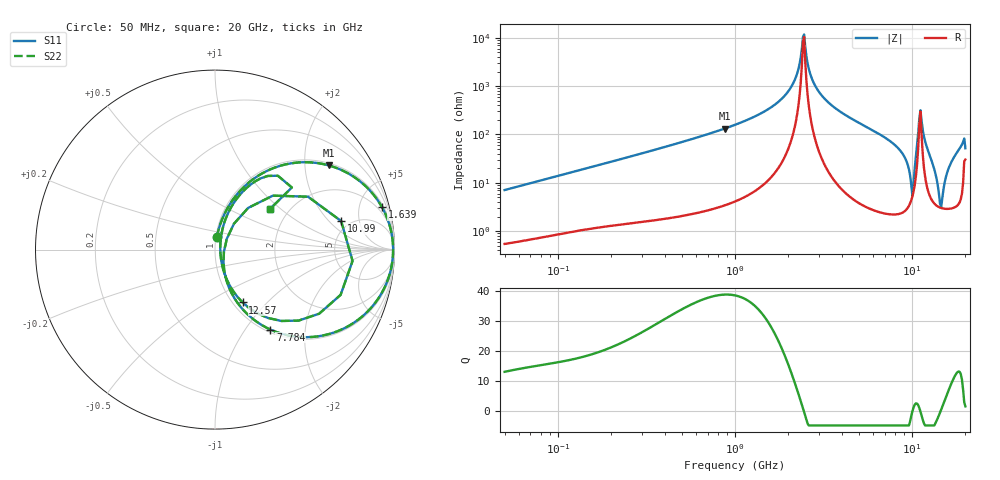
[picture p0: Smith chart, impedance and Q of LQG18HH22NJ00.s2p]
!Murata Part Number: LQG18HH22NJ00
!These Parameters are Measured in Series Mode Connection
!  o--[Z]--o
!Port1  Port2
!  o-------o
!Freq. Start=50[MHz] Stop=20[GHz], 401[Steps]
# Hz S RI R 50
!Freq.(Hz) S11(Real) S11(Imag) S21(Real) S21(Imag) S12(Real) S12(Imag) S22(Real) S22(Imag)
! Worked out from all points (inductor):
!   401 points, 50 MHz to 20 GHz, reference 50 ohm
!   read as one part in series: L = 22.4 nH near 51.52 MHz
!   highest Q = 38.9 at 873.9 MHz (marker M1), where L = 24.1 nH
!   self-resonance near 2.42 GHz
!   S11 on the Smith chart (normalised r, x): 50 MHz: 1.01, +0.14; 1.639 GHz: 1.29, +7.77; 7.784 GHz: 1.04, -1.32; 10.99 GHz: 4.23, +2.80; 12.57 GHz: 1.11, -0.73; 20 GHz: 1.61, +0.84
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5e7  0.0103 0.0696  0.9897 -0.0696  0.9897 -0.0696  0.0103 0.0696
1.364002e8  0.0434 0.1778  0.9566 -0.1778  0.9566 -0.1778  0.0434 0.1778
3.721004e8  0.2145 0.3939  0.7855 -0.3939  0.7855 -0.3939  0.2145 0.3939
8.738837e8  0.6342 0.469  0.3658 -0.469  0.3658 -0.469  0.6342 0.469
1e9  0.7106 0.4407  0.2894 -0.4407  0.2894 -0.4407  0.7106 0.4407
1.639343e9  0.9302 0.2369  0.0698 -0.2369  0.0698 -0.2369  0.9302 0.2369
2.114743e9  0.9839 0.0896  0.0161 -0.0896  0.0161 -0.0896  0.9839 0.0896
2.419936e9  0.9924 0.00573  0.00763 -0.00573  0.00763 -0.00573  0.9924 0.00573
2.493527e9  0.9923 -0.0132  0.00773 0.0132  0.00773 0.0132  0.9923 -0.0132
2.728004e9  0.9875 -0.0705  0.0125 0.0705  0.0125 0.0705  0.9875 -0.0705
3.792786e9  0.9067 -0.2771  0.0933 0.2771  0.0933 0.2771  0.9067 -0.2771
7.442007e9  0.3623 -0.4659  0.6377 0.4659  0.6377 0.4659  0.3623 -0.4659
7.784049e9  0.3085 -0.4454  0.6915 0.4454  0.6915 0.4454  0.3085 -0.4454
9.041845e9  0.1254 -0.2964  0.8746 0.2964  0.8746 0.2964  0.1254 -0.2964
1.004137e10  0.0497 -0.0118  0.9503 0.0118  0.9503 0.0118  0.0497 -0.0118
1.066139e10  0.3225 0.3007  0.6775 -0.3007  0.6775 -0.3007  0.3225 0.3007
1.098561e10  0.7029 0.159  0.2971 -0.159  0.2971 -0.159  0.7029 0.159
1.166392e10  0.4652 -0.3957  0.5348 0.3957  0.5348 0.3957  0.4652 -0.3957
1.257102e10  0.154 -0.2945  0.846 0.2945  0.846 0.2945  0.154 -0.2945
1.460232e10  0.0293 0.009  0.9707 -0.009  0.9707 -0.009  0.0293 0.009
1.670968e10  0.0923 0.2403  0.9077 -0.2403  0.9077 -0.2403  0.0923 0.2403
2e10  0.3052 0.225  0.6948 -0.225  0.6948 -0.225  0.3052 0.225
